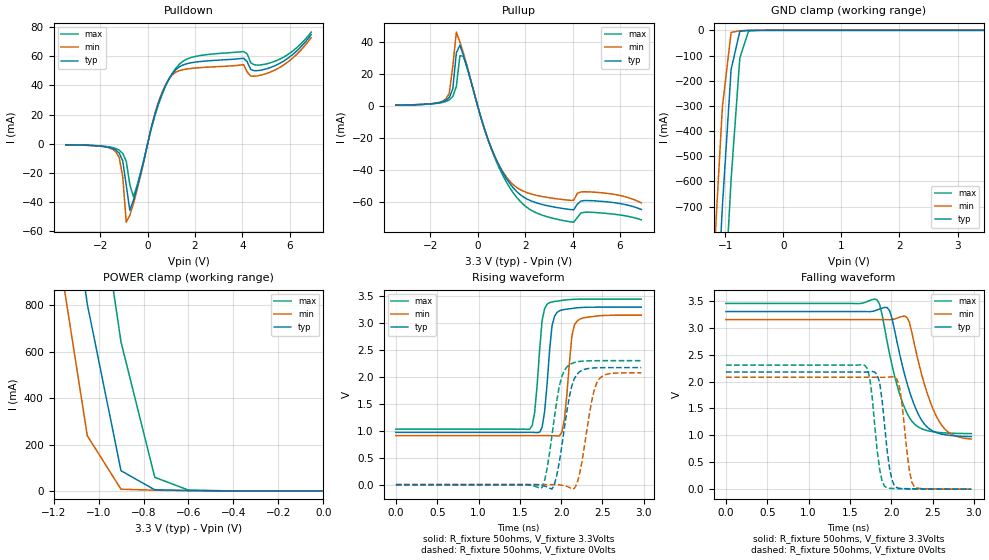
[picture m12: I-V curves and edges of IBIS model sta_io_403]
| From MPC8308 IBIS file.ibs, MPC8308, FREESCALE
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[Model]   sta_io_403   |
Model_type   I/O
Vinl = 0.8
Vinh = 2
Vmeas = 1.65
Cref = 5E-11
Rref = 50
Vref = 0
| variable   typ   min   max
C_comp   494.81f   465.60f   523.27f
[Model Spec]
| subparameter   typ   min   max
S_overshoot_high  3.300   3.135   3.465
S_overshoot_low   -200.00m  -100.00m  -300.00m
D_overshoot_high  4.000   4.000   4.000
D_overshoot_low   -1.000   -1.000   -1.000
D_overshoot_time  1.000n   1.000n   1.000n
| variable   typ   min   max
[Temperature Range]   55.0   110.0   0.0
| variable   typ   min   max
[Pullup Reference]   3.300V   3.150V   3.450V
| variable   typ   min   max
[Pulldown Reference]   0.000V   0.000V   0.000V
| variable   typ   min   max
[POWER_Clamp_Reference]   3.300V   3.150V   3.450V
| variable   typ   min   max
[GND_Clamp_Reference]   0.000V   0.000V   0.000V
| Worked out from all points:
|   slope of the pulldown table from 0 to 0.495 V, typ, clamps not added: 16.8 ohm
|   slope of the pullup table from 0 to 0.495 V, typ, clamps not added: 21.4 ohm
|   GND clamp passes 1 mA (typ) near -0.62 V on its own axis
|   POWER clamp passes 1 mA (typ) near -0.51 V on its own axis
|   rising waveform, R_fixture 50ohms, V_fixture 3.3Volts: 20-80 % time 77.3ps typ, 77.7ps min, 75.6ps max; typ from 0.972 V to 3.3 V
|   rising waveform, R_fixture 50ohms, V_fixture 0Volts: 20-80 % time 135ps typ, 136ps min, 133ps max; typ from 0 V to 2.18 V
|   falling waveform, R_fixture 50ohms, V_fixture 3.3Volts: 20-80 % time 256ps typ, 262ps min, 237ps max; typ from 3.3 V to 0.977 V
|   falling waveform, R_fixture 50ohms, V_fixture 0Volts: 20-80 % time 93.8ps typ, 90.9ps min, 93.9ps max; typ from 2.18 V to 0 V
[Pulldown]
| pulldown in the table = pulldown subtract gnd_clamp
|Voltage   I(typ)   I(min)   I(max)
-3.45V    -644.6uA   -622.1uA   -626.2uA
-1.35V    -4.132mA   -5.207mA   -3.151mA
-1.05V    -11.56mA   -22.33mA   -6.546mA
-900mV    -28.51mA   -53.69mA   -11.94mA
-750mV    -45.44mA   -48.92mA   -27.87mA
-600mV    -38.8mA    -41.13mA   -36.25mA
300mV     19.54mA    20.42mA    18.85mA
1.05V     48.13mA    47.36mA    48.56mA
2.85V     57.21mA    52.8mA     61.7mA
4.05V     58.64mA    54.24mA    63.22mA
4.8V      50.53mA    47.13mA    54.12mA
6.9V      74.81mA    72.75mA    76.56mA
[Pullup]
| pullup in the table = pullup subtract power_clamp
|Voltage   I(typ)   I(min)   I(max)
-3.45V    575.1uA    552.8uA    582.1uA
-1.35V    3.502mA    4.354mA    2.812mA
-1.2V     5.372mA    7.941mA    3.847mA
-1.05V    10.7mA     24.78mA    5.99mA
-900mV    33.33mA    46.38mA    12.23mA
-750mV    38.18mA    40.15mA    31.61mA
-600mV    31.6mA     33.17mA    31.19mA
450mV     -21.33mA   -21.71mA   -21.74mA
1.5V      -51.28mA   -49.3mA    -54.43mA
3.45V     -63.9mA    -58.36mA   -71.31mA
4.65V     -59.24mA   -53.78mA   -66.52mA
6.9V      -64.85mA   -60.73mA   -71.31mA
[GND_clamp]
|Voltage   I(typ)   I(min)   I(max)
-3.45V    -12.31A    -11.88A    -12.85A
-1.2V     -1.358A    -924.9mA   -1.906A
-1.05V    -698.5mA   -303.5mA   -1.226A
-900mV    -155.7mA   -8.533mA   -591.6mA
-750mV    -3.954mA   -1.306mA   -110.3mA
-600mV    -606.2uA   -198.8uA   -3.05mA
-300mV    -1.971uA   -109.9nA   -16.38uA
3.45V     171.4nA    873.4nA    35.1nA
[POWER_clamp]
|Voltage   I(typ)   I(min)   I(max)
-3.3V     18.63A     17.95A     19.5A
-1.2V     1.853A     1.171A     2.731A
-1.05V    806.1mA    238.2mA    1.631A
-900mV    87.08mA    7.341mA    642.4mA
-750mV    4.847mA    3.182mA    58.69mA
-600mV    1.868mA    967.7uA    3.546mA
0V        962.3pA    16.62pA    35.1nA
[Ramp]
|Voltage   I(typ)   I(min)   I(max)
dV/dt_f   1.44/358.343p 1.39/371.244p 1.50/332.583p
dV/dt_r   1.33/186.790p 1.28/189.492p 1.41/182.681p
R_load=50ohms
| R_load was connected to ground for Ramp_up test and power for Ramp_dn test
[Rising_Waveform]
R_fixture=50ohms
V_fixture=3.3Volts
V_fixture_min=3.15Volts
V_fixture_max=3.45Volts
|C_fixture=1E-15f
|L_fixture=1E-15h
|C_dut=1E-15fh
|R_dut=0.001ohm
|L_dut=1E-12h
|time   V(typ)   V(min)   V(max)
0s        972mV      911mV      1.031V
1.62ns    973mV      911mV      1.031V
1.68ns    971mV      911mV      1.348V
1.74ns    976mV      911mV      2.512V
1.8ns     1.356V     912mV      3.273V
1.89ns    2.958V     911mV      3.397V
1.98ns    3.233V     908mV      3.418V
2.13ns    3.275V     2.759V     3.443V
2.19ns    3.286V     3.034V     3.447V
2.97ns    3.3V       3.15V      3.45V
[Rising_Waveform]
R_fixture=50ohms
V_fixture=0Volts
|C_fixture=1E-15f
|L_fixture=1E-15h
|C_dut=1E-15fh
|R_dut=0.001ohm
|L_dut=1E-12h
|time   V(typ)   V(min)   V(max)
0s        0V         0V         0V
1.77ns    -17mV      0V         -54mV
1.83ns    -41mV      0V         298mV
1.92ns    13mV       1mV        1.268V
2.01ns    735mV      -11mV      2.019V
2.1ns     1.637V     -52mV      2.228V
2.16ns    1.972V     -70mV      2.271V
2.22ns    2.095V     176mV      2.29V
2.43ns    2.172V     1.886V     2.304V
2.97ns    2.176V     2.079V     2.305V
[Falling_Waveform]
R_fixture=50ohms
V_fixture=3.3Volts
V_fixture_min=3.15Volts
V_fixture_max=3.45Volts
|C_fixture=1E-15f
|L_fixture=1E-15h
|C_dut=1E-15fh
|R_dut=0.001ohm
|L_dut=1E-12h
|time   V(typ)   V(min)   V(max)
0s        3.3V       3.15V      3.45V
1.83ns    3.33V      3.15V      3.515V
1.89ns    3.363V     3.15V      3.239V
1.98ns    3.317V     3.148V     2.515V
2.16ns    2.143V     3.217V     1.518V
2.22ns    1.823V     3.102V     1.33V
2.34ns    1.356V     2.298V     1.145V
2.55ns    1.049V     1.345V     1.058V
2.7ns     1.001V     1.05V      1.041V
2.97ns    977mV      932mV      1.032V
[Falling_Waveform]
R_fixture=50ohms
V_fixture=0Volts
|C_fixture=1E-15f
|L_fixture=1E-15h
|C_dut=1E-15fh
|R_dut=0.001ohm
|L_dut=1E-12h
|time   V(typ)   V(min)   V(max)
0s        2.176V     2.079V     2.305V
1.68ns    2.175V     2.079V     2.3V
1.74ns    2.181V     2.079V     2.072V
1.86ns    1.979V     2.078V     377mV
1.98ns    386mV      2.083V     17mV
2.04ns    61mV       2.083V     11mV
2.1ns     17mV       1.903V     8mV
2.22ns    8mV        348mV      4mV
2.28ns    6mV        44mV       3mV
2.97ns    0V         0V         0V
